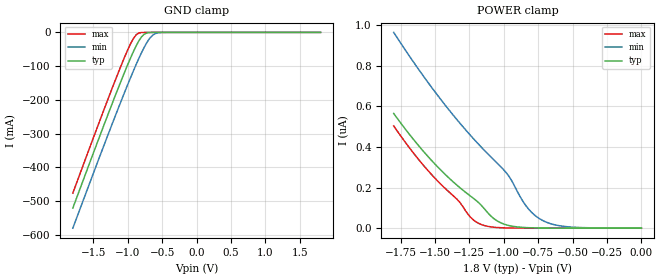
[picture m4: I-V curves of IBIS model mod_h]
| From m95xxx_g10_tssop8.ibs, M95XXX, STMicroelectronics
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|   Model mod_h
[Model]   mod_h
Model_type Input
Vinl   =   0.540V
Vinh   =   1.260V
C_comp   2.120pF   2.024pF   2.323pF
[Temperature Range]  25.0000   0.1050k   -40.0000
[Voltage Range]   1.8000V   1.7000V   2.0000V
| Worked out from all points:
|   GND clamp passes 1 mA (typ) near -0.70 V on its own axis
[GND_clamp]
|Voltage   I(typ)   I(min)   I(max)
-1.8V     -520.9mA   -580.3mA   -476.5mA
-1.2V     -196.3mA   -256.7mA   -150.7mA
-1.04V    -114.2mA   -173.8mA   -69.64mA
-960mV    -75.5mA    -133.8mA   -33.44mA
-880mV    -40.19mA   -95.27mA   -7.262mA
-800mV    -12.93mA   -59.44mA   -437.7uA
-760mV    -5.115mA   -43.21mA   -157.1uA
-720mV    -1.572mA   -28.76mA   -100.4uA
-640mV    -131.4uA   -8.363mA   -67.87uA
-560mV    -23uA      -1.269mA   -44.38uA
-480mV    -5.764uA   -149uA     -22.96uA
1.8V      15.18pA    369.3pA    13.84pA
[POWER_clamp]
|Voltage   I(typ)   I(min)   I(max)
-1.8V     565.1nA    965nA      503.9nA
-1.64V    423.8nA    803nA      356.1nA
-1.5V     315.7nA    671.8nA    246.1nA
-1.34V    211.6nA    534.4nA    142.5nA
-1.2V     135.9nA    425.9nA    30.17nA
-1.08V    51.18nA    341.5nA    5.039nA
-1.02V    25.67nA    301.1nA    1.994nA
-960mV    12.45nA    253.1nA    793.5pA
-840mV    2.77nA     111.4nA    147.1pA
-760mV    1.008nA    55.69nA    65.8pA
-560mV    102.4pA    8.462nA    36.58pA
0V        25.78pA    670.7pA    28.23pA
